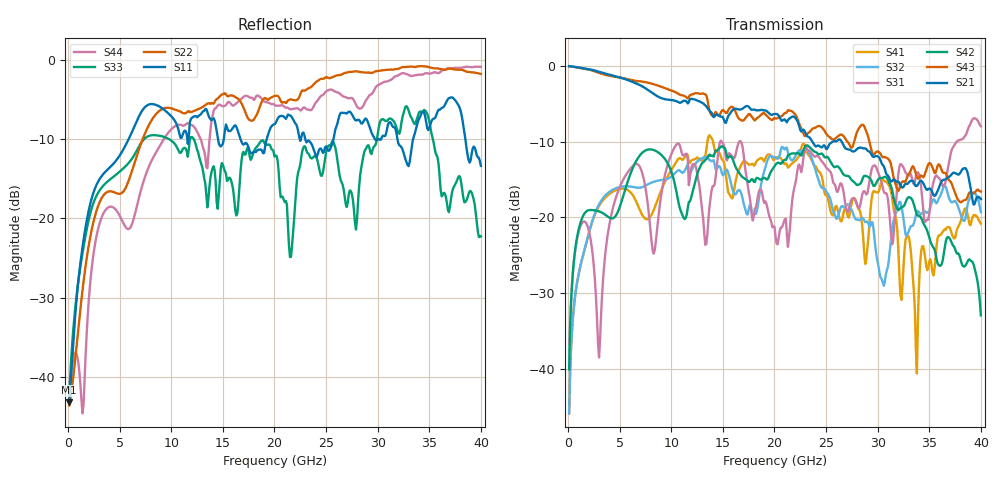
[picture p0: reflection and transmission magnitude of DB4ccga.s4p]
! ADC12DJ3200QML-SP
! 196-pin NWE package
! CCGA Ceramic Package with columns (ceramic column grid array)
! Texas Instruments 4/21/2021
! Single-ended  S-parameters
! PORT#  PORT_NAME  NET_NAME
! PORT1:  DAxN.DIEBUMP DAxN
! PORT2:  DAxN.BGA  DAxN
! PORT3:  DAxP.DIEBUMP DAxP
! PORT4:  DAxP.BGA  DAxP
! Touchstone Ver. 1.0
! Number of ports is 4
# Hz	S	MA	R	50.000000
! SCATTERING PARAMETERS  :
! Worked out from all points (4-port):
!   400 points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, 100 MHz to 40 GHz, reference 50 ohm
!   strongest paths, dB at 100 MHz, 10.1 GHz, 20.1 GHz, 30.1 GHz, 40 GHz:
!     S21: -0.1, -4.5, -6.4, -12.0, -17.6
!     S43: -0.1, -3.3, -7.0, -11.4, -16.6
!     S42: -40.1, -14.4, -13.1, -14.9, -32.9
!     S31: -40.0, -11.4, -22.5, -14.2, -8.0
!     S32: -45.8, -14.5, -12.1, -26.6, -19.3
!     S41: -45.8, -13.5, -12.2, -16.6, -20.8
!   lowest |S11| = -43.2 dB at 100 MHz (marker M1), VSWR 1.01, Z = 50.7 - j0.0387 ohm
!   |S11| at or under -10 dB: start of sweep to 5.874 GHz; 16.7 GHz to 19.25 GHz (2.548 GHz wide, 14.2 % of centre); 22.98 GHz to 25.72 GHz (2.735 GHz wide, 11.2 % of centre)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
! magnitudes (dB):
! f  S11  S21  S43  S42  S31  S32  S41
! 100 MHz  -43.2  -0.1  -0.1  -40.1  -40.0  -45.8  -45.8
! 2.6 GHz  -16.2  -0.6  -0.8  -19.1  -28.3  -19.5  -19.6
! 7.7 GHz  -5.7  -3.2  -2.2  -11.1  -18.0  -15.7  -20.2
! 21.6 GHz  -7.1  -6.8  -6.0  -11.6  -19.4  -12.4  -13.0
! 30.5 GHz  -9.6  -13.1  -12.1  -14.8  -16.1  -28.6  -15.0
! 33.8 GHz  -8.2  -15.9  -14.7  -19.6  -14.1  -19.3  -40.6
! 40 GHz  -13.4  -17.6  -16.6  -32.9  -8.0  -19.3  -20.8
